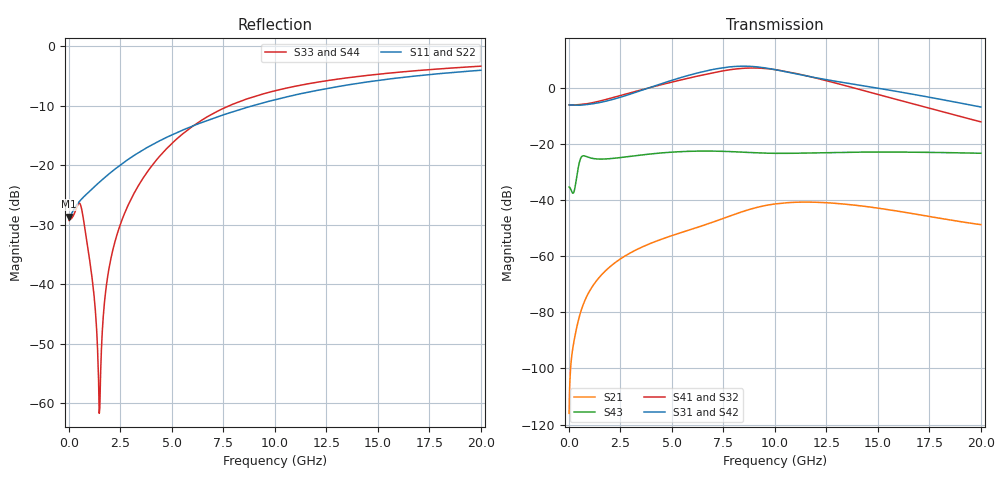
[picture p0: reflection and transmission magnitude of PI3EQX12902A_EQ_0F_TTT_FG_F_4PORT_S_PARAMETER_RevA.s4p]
! NPort=4 DATA=2000 NOISE=0 GROUPDELAY=0 COMPLEX_DATAFORMAT=POLAR
! NumOfBlock=1 NumOfParam=0
! .MODEL Smodel S TSTONEFILE=PI3EQX12902A_EQ_0F_TTT_FG_F_4PORT_S_PARAMETER_RevA.s4p TYPE=S
!  -- The above .MODEL line can be used for the S element in the netlist.
! The s parameter is extracted from the linear redriver, it is not bi-directional; only s(4,1)s(4,2) and s(3,1)s(3,2)
! should be the insertion loss
!Port definition:
!Port1 = input+
!Port2 = input-
!Port3 = output+
!Port4 = output-
# Hz S MA R  50
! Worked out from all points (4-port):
!   2000 points, 10 MHz to 20 GHz, reference 50 ohm
!   strongest paths, dB at 10 MHz, 5.01 GHz, 10.01 GHz, 15.01 GHz, 20 GHz:
!     S31: -6.0, 2.7, 6.5, -0.1, -6.8
!     S42: -6.0, 2.6, 6.3, -0.3, -7.0
!     S41: -6.0, 2.1, 6.5, -2.3, -12.1
!     S32: -6.0, 2.1, 6.5, -2.4, -12.2
!     S43: -35.3, -22.9, -23.3, -22.9, -23.3
!     S21: -116.0, -52.6, -41.4, -42.9, -48.7
!   lowest |S11| = -28.6 dB at 10 MHz (marker M1), VSWR 1.08, Z = 46.4 - j0.0607 ohm
!   |S11| at or under -10 dB: start of sweep to 8.925 GHz
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1e7  0.03704 -179.0  1.583e-06 51.7  0 0.0  0 0.0
     1.583e-06 51.7  0.03704 -179.0  0 0.0  0 0.0
     0.4985 -0.1  0.4985 179.9  0.03429 6.0  0.01709 -177.1
     0.4985 179.9  0.4985 -0.1  0.01709 -177.1  0.03429 6.0
1.49e9  0.0722 -133.4  0.0004263 115.5  3.743e-09 177.1  5.623e-09 -173.9
        0.0004263 115.5  0.0722 -133.4  5.625e-09 -173.8  3.744e-09 177.2
        0.5483 6.0  0.5842 179.7  0.0008858 -60.3  0.05389 -174.9
        0.5824 179.6  0.5482 5.7  0.05389 -174.8  0.0009453 -62.8
6.19e9  0.2196 -112.2  0.003224 80.8  1.928e-06 -28.7  1.191e-06 82.4
        0.003227 80.8  0.2196 -112.2  1.199e-06 82.7  1.922e-06 -28.6
        1.826 -44.4  1.609 104.9  0.2235 -48.5  0.07424 142.5
        1.607 105.0  1.796 -45.0  0.07464 142.6  0.2228 -48.5
7.87e9  0.2784 -112.1  0.005276 67.6  6.121e-06 -78.1  3.876e-06 39.8
        0.005292 67.6  0.2784 -112.1  3.918e-06 39.8  6.113e-06 -78.0
        2.382 -89.1  2.122 58.2  0.3211 -64.9  0.07268 125.1
        2.121 58.4  2.339 -89.6  0.07315 125.1  0.3204 -64.8
9.41e9  0.3338 -113.4  0.007797 43.4  1.185e-05 -123.9  8.553e-06 -11.2
        0.007833 43.3  0.3338 -113.4  8.652e-06 -11.4  1.184e-05 -123.8
        2.306 -135.0  2.235 6.4  0.3963 -77.2  0.06865 113.8
        2.235 6.5  2.263 -135.5  0.06903 113.6  0.3959 -77.1
1.178e10  0.4159 -116.9  0.009161 0.0  2.084e-05 -178.0  1.513e-05 -86.9
          0.009201 -0.4  0.4159 -116.9  1.529e-05 -87.3  2.08e-05 -178.0
          1.566 172.2  1.559 -66.0  0.4892 -91.7  0.06922 100.4
          1.564 -65.7  1.528 171.8  0.06934 100.1  0.4894 -91.6
2e10  0.6277 -131.5  0.003753 -67.6  4.558e-05 49.5  1.719e-05 109.9
      0.003656 -68.1  0.6278 -131.5  1.734e-05 109.0  4.54e-05 49.7
      0.4567 48.0  0.2443 139.2  0.6794 -119.6  0.06848 46.2
      0.2483 138.9  0.4465 48.5  0.06843 46.2  0.6798 -119.6
